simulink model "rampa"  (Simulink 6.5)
settings: Solver=FixedStepDiscrete  StartTime=0.0  StopTime=20e-6  RelTol=1e-6
undefined symbols (not defined in the file or in its folder): blocks, Discrete, interp1, powergui, ZData
libraries: powerlib x6

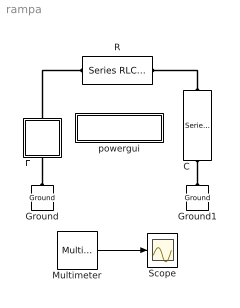
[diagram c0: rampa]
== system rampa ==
  C : powerlib/Elements/Series RLC Branch  Orientation=down  DialogController=PMDialogs.PMDefaultMaskDlg  PhysicalDomain=powersysdomain  SubClassName=unknown  LeftPortType=p1  RightPortType=p1  LConnTagsString=__new0  RConnTagsString=__new0  BranchType=C  Resistance=1  Inductance=1e-3  SetiL0=off  InitialCurrent=0  Capacitance=10e-9  Setx0=on  InitialVoltage=0  Measurements=Branch voltage
  E : Subsystem  Orientation=up  mask(Proizvolen generator){vreme=[0	5	20]/1e6, napon=[0	100 100]*1000}
      mask prompts: vreme "Vreme (s)"; napon "Napon (V)"
      mask help: So ovoj element e definiran idealen naponski generator so proizvolen oblik. Oblikot na naponot se definira so pomos na dva vektori, pri sto vo prviot vektor se dadeni diskretni vremenski momenti dodeka vrednostite na naponot vo tie momenti se dadeni vo vtoriot vektor. Za ostanatite vremenski momenti koi sto ne se dadeni vo vektorite modelot pravi linearna interpolacija.
  Ground : powerlib/Elements/Ground  Orientation=down  DialogController=PMDialogs.PMDefaultMaskDlg  PhysicalDomain=powersysdomain  SubClassName=unknown  LeftPortType=p1  RightPortType=p1  LConnTagsString=a
  Ground1 : powerlib/Elements/Ground  Orientation=down  DialogController=PMDialogs.PMDefaultMaskDlg  PhysicalDomain=powersysdomain  SubClassName=unknown  LeftPortType=p1  RightPortType=p1  LConnTagsString=a
  Multimeter : powerlib/Measurements/Multimeter  SystemSampleTime=-1  PhasorSimulation=off  OutputType=Complex  sel=[1 2]  L=2  Gain=[1 1]  yselected={'Ub: C','Usrc: E/Kontrolirano E'};  PSBOutputType=1  PSBequivalent=0  AxesSetting=[0,0.1,-100,100]  Display=0  SavedBlockNames=-11
  R : powerlib/Elements/Series RLC Branch  DialogController=PMDialogs.PMDefaultMaskDlg  PhysicalDomain=powersysdomain  SubClassName=unknown  LeftPortType=p1  RightPortType=p1  LConnTagsString=__new0  RConnTagsString=__new0  BranchType=R  Resistance=100  Inductance=1e-3  SetiL0=on  InitialCurrent=0  Capacitance=1e-6  Setx0=off  InitialVoltage=0  Measurements=None
  Scope : Scope
  powergui : Subsystem  AncestorBlock=powerlib/powergui  InitFcn=powergui( 'InitFcn_Callback' , gcb , 0 , [ ] );  mask(PSB option menu block){SimulationMode=Discrete, SampleTime=0.01e-6, echomessages=off, RestoreLinks=warning, x0status=blocks, Frange=[0:2:500], Ylog=off, Xlog=on, ShowGrid=off, save=off, variable=ZData, structure=, ZoomFFT=on, StartTime=0.0, cycles=1, DisplayStyle=1, fundamental=60, FreqAxis=off, MaxFrequency=1000, frequencyindice=0, frequencyindicesteady=1, RmsSteady=1, display=off, Ts=0, frequency=60, methode=off, HookPort=off, Interpol=off}
      mask prompts: SimulationMode "Simulation mode"; SampleTime "Sample time Ts (when simulation mode is Discrete) (s)"; echomessages "Echo  Messages"; RestoreLinks "Restore disabled links"; x0status "Initial electrical states status"; Frange "Impedance tool: Frequency Range"; Ylog "Impedance tool: Log impedance"; Xlog "Impedance tool: log Frequency"; ShowGrid "Impedance tool: grid"; save "Impedance tool: Save Data To Workspace"; variable "Impedance tool: Variable Name"; structure "Structure Name (PSBFFTSCOPE)"; ZoomFFT "ZoomFFT (PSBFFTSCOPE)"; StartTime "Start Time (PSBFFTSCOPE)"; cycles "Cycles (PSBFFTSCOPE)"; DisplayStyle "Display style (PSBFFTSCOPE)"; fundamental "Fundamental (PSBFFTSCOPE)"; FreqAxis "Frequency Axis (PSBFFTSCOPE)"; MaxFrequency "Max Frequency (PSBFFTSCOPE)"; frequencyindice "Load flow frequency (Hz)"; frequencyindicesteady "Frequency indice (STEADYSTATE)"; RmsSteady "RMS display (STEADYSTATE)"; display "Display Results"; Ts "OBSOLETE 1"; frequency "Phasor frequency (Hz)"; methode "Phasor simulation"; HookPort "Hook port"; Interpol "Interpolate"
      mask init:
      | powerlibroot = which('powersysdomain');
      | PSBroot = powerlibroot(1:end-16);
      | %
      | switch SimulationMode
      | 	case 1
      | 		message=sprintf('Continuous');
      | 	case 2
      |         SampleTimeeval=evalin('base',SampleTime,'NaN');
      |         if isnan(SampleTimeeval)
      |             message=sprintf('Warning !!,\nUndefined sample time');
      |         else
      |             message=sprintf('Discrete,\nTs = %.4g s.',SampleTimeeval);
      |         end
      | 	case 3
      | 		message=sprintf('Phasors');
      | end
      | if strcmp(bdroot,'powerlib')
      |   message='powergui';
      | end
      | power_initmask();
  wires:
  Multimeter/1 -> Scope/1
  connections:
  C/LConn1 -- R/RConn1
  Ground1/LConn1 -- C/RConn1
  Ground/LConn1 -- E/LConn1
  E/RConn1 -- R/LConn1

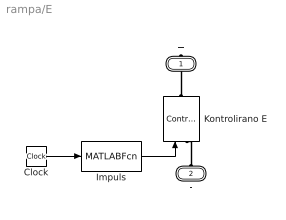
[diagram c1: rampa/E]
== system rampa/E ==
  Clock : Clock
  Impuls : MATLABFcn  MATLABFcn=interp1(vreme, napon, u)  OutputSignalType=real
  Kontrolirano E : powerlib/Electrical Sources/Controlled Voltage Source  Orientation=up  DialogController=PMDialogs.PMDefaultMaskDlg  SystemSampleTime=-1  Initialize=on  Source_Type=AC  Amplitude=0  Phase=0  Frequency=0  Measurements=Voltage
  + : PMIOPort  Orientation=down  Port=1  Side=Right
  - : PMIOPort  Orientation=up  Port=2  Side=Left
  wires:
  Impuls/1 -> Kontrolirano E/1
  Clock/1 -> Impuls/1
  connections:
  +/RConn1 -- Kontrolirano E/RConn1
  -/RConn1 -- Kontrolirano E/LConn1

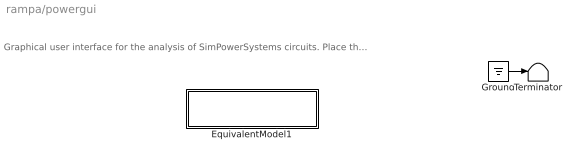
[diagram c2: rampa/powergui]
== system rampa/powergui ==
  note: Graphical user interface for the analysis of SimPowerSystems circuits. Place the Powergui block in the top-level of your model and double-click on it to open the GUI.
  EquivalentModel1 : Subsystem
  Ground : Ground
  Terminator : Terminator
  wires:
  Ground/1 -> Terminator/1

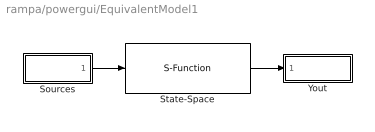
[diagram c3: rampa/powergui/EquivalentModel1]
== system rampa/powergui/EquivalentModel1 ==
  Sources : Subsystem
  State-Space : S-Function  FunctionName=sfun_spssw_discc  Parameters=Ts,A, B, C, D, x0
  Yout : Subsystem
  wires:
  Sources/1(u) -> State-Space/1
  State-Space/1 -> Yout/1(v,i)

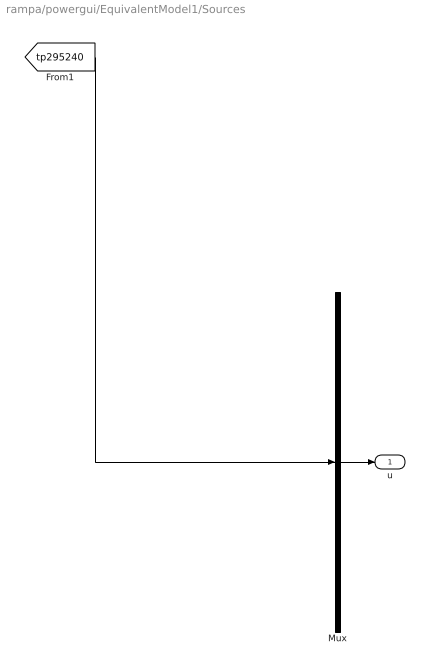
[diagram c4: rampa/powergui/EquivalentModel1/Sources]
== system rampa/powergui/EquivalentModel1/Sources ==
  Mux : Mux  Inputs=1
  u : Outport
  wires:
  Mux/1 -> u/1
  [tp295240] -> Mux/1

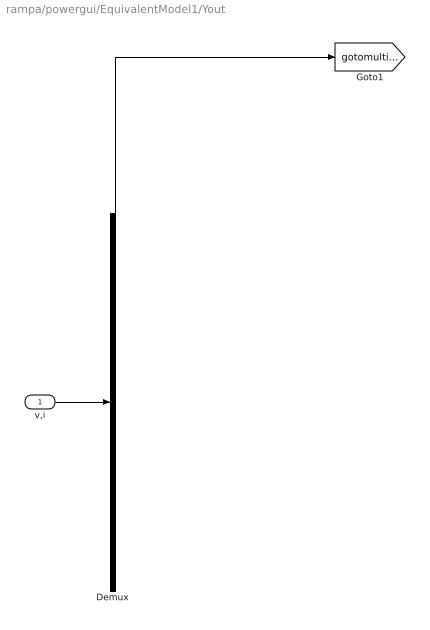
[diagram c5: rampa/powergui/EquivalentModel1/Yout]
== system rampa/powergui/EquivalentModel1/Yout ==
  v,i : Inport
  Demux : Demux  Outputs=1
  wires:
  v,i/1 -> Demux/1
  Demux/1 -> [gotomultimeterPSB]
